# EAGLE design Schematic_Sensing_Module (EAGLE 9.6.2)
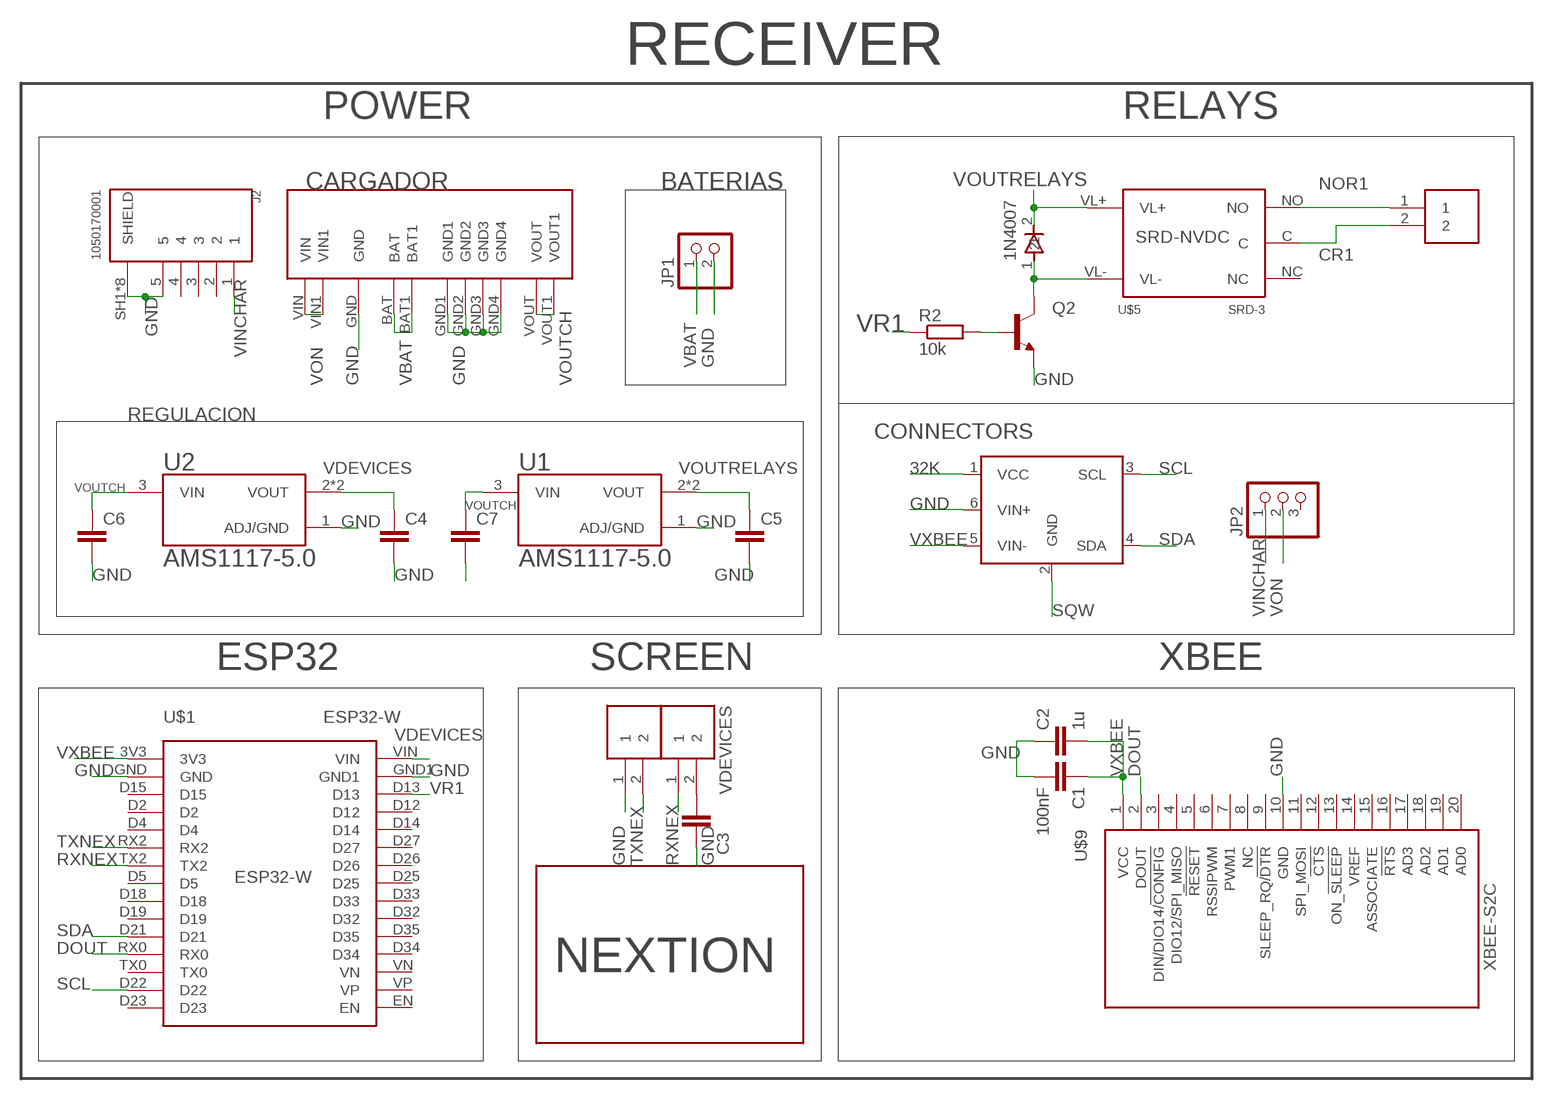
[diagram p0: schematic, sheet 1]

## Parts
1N4007  1N4007SMA  [SMA]
C1  100nF  C-EUC1206  [C1206]
C2  1u  C-EUC1206  [C1206]
C3  100nF  C-EUC1206  [C1206]
C4  C-EUC1206  [C1206]
C5  C-EUC1206  [C1206]
C6  C-EUC1206  [C1206]
C7  C-EUC1206  [C1206]
CARGADOR  MODULO_CARGA_5V  [MODULO_CARGA_5V]
CONN1  TERMINAL-TB2  [TERMINAL-TB2]
CONN2  TERMINAL-TB2  [TERMINAL-TB2]
J2  1050170001  [MOLEX_1050170001]
JP1  PINHD-1X2  [1X02]
JP2  PINHD-1X3  [1X03]
Q2  MMBT2222A  [SOT23]
R2  10k  R-EU_R1206  [R1206]
REL1  TERMINAL-TB2  [TERMINAL-TB2]
U1  AMS1117-5.0  [SOT229P700X180-4N]
U2  AMS1117-5.0  [SOT229P700X180-4N]
U$1  ESP32-W  [DIP]
U$2  NX4024T032  [NX4024T032]
U$3  INABB  [INA219-MODULE]
U$5  SRD-3  [SRD-N]
U$9  XBEE-S2C  [XBEE-DIP]

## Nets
32K: U$3.1(VCC)
CR1: REL1.2 U$5.C
DOUT: U$1.RX0 U$9.2(DOUT)
GND: C1.2 C2.1 C3.2 C4.2 C5.2 C6.2 C7.2 CARGADOR.GND CARGADOR.GND1 CARGADOR.GND2 CARGADOR.GND3 CARGADOR.GND4 CONN1.1 J2.5 J2.SH1(SHIELD) J2.SH2(SHIELD) J2.SH3(SHIELD) J2.SH4(SHIELD) J2.SH5(SHIELD) J2.SH6(SHIELD) J2.SH7(SHIELD) J2.SH8(SHIELD) JP1.2 Q2.2(E) U1.1(ADJ/GND) U2.1(ADJ/GND) U$1.GND U$1.GND1 U$3.6(VIN+) U$9.10(GND)
N$5: Q2.1(B) R2.2
N$8: 1N4007.1 Q2.3(C) U$5.VL-
NOR1: REL1.1 U$5.NO
RXNEX: CONN2.1 U$1.TX2
SCL: U$1.D22 U$3.3(SCL)
SDA: U$1.D21 U$3.4(SDA)
SQW: U$3.2(GND)
TXNEX: CONN1.2 U$1.RX2
VBAT: CARGADOR.BAT CARGADOR.BAT1 JP1.1
VDEVICES: C3.1 C4.1 CONN2.2 U2.2(VOUT) U2.4(VOUT) U$1.VIN
VINCHAR: J2.1 JP2.1
VON: CARGADOR.VIN CARGADOR.VIN1 JP2.2
VOUTCH: C6.1 C7.1 CARGADOR.VOUT CARGADOR.VOUT1 U1.3(VIN) U2.3(VIN)
VOUTRELAYS: 1N4007.2 C5.1 U1.2(VOUT) U1.4(VOUT) U$5.VL+
VR1: R2.1 U$1.D13
VXBEE: C1.1 C2.2 U$1.3V3 U$3.5(VIN-) U$9.1(VCC)
Unconnected: J2.2 J2.3 J2.4 JP2.3 U$1.D2 U$1.D4 U$1.D5 U$1.D12 U$1.D14 U$1.D15 U$1.D18 U$1.D19 U$1.D23 U$1.D25 U$1.D26 U$1.D27 U$1.D32 U$1.D33 U$1.D34 U$1.D35 U$1.EN U$1.TX0 U$1.VN U$1.VP U$5.NC U$9.3(DIN/DIO14/!CONFIG) U$9.4(DIO12/SPI_MISO) U$9.5(!RESET) U$9.6(RSSIPWM) U$9.7(PWM1) U$9.8(NC) U$9.9(SLEEP_RQ/!DTR) U$9.11(SPI_MOSI) U$9.12(!CTS) U$9.13(ON_!SLEEP) U$9.14(VREF) U$9.15(ASSOCIATE) U$9.16(!RTS) U$9.17(AD3) U$9.18(AD2) U$9.19(AD1) U$9.20(AD0)

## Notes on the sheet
- RECEIVER
- POWER | RELAYS
- BATERIAS
- REGULACION
- CONNECTORS
- ESP32 | SCREEN | XBEE

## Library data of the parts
1N4007 = 1n400X:1N4007SMA
C1-C7 = rcl:C-EU: CAPACITOR, European symbol; SPICEPREFIX: C
CARGADOR = Modulo_Carga:MODULO_CARGA_5V
CONN1 CONN2 REL1 = TERMINAL-TB001:TERMINAL-TB2
J2 = 1050170001_MOLEX:1050170001: Conn.; Data; USB; Recept.; Micro; B Type; Bottom Mount, SMT, with Solder Tabs, Lead-Free Check prices; AVAILABILITY: Warning; DESCRIPTION: USB - micro B USB 2.0 Receptacle Connector 5 Position Surface Mount, Right Angle; Through Hole; MF: Molex; MP: 1050170001; PACKAGE: None; PRICE: None; PURCHASE-URL: https://pricing.snapeda.com/search/part/1050170001/?ref=eda
JP1 = pinhead:PINHD-1X2: PIN HEADER
JP2 = pinhead:PINHD-1X3: PIN HEADER
Q2 = MMBT2222A:MMBT2222A: 2N2222 General Purpose NPN Transistor Check prices; AVAILABILITY: Good; DESCRIPTION: Bipolar (BJT) Transistor NPN 40V 600mA 300MHz 225mW Surface Mount SOT-23; MF: ON Semiconductor; MP: MMBT2222A; PACKAGE: None; PRICE: None
R2 = rcl:R-EU_: RESISTOR, European symbol; SPICEPREFIX: R
U1 U2 = AMS1117-5.0:AMS1117-5.0: Sot223/Pkg 1-Amp 5-Volt Low Drop Out Voltage Regulatator; AVAILABILITY: Unavailable; DESCRIPTION: Sot223/Pkg 1-Amp 5-Volt Low Drop Out Voltage Regulatator; MF: Advanced Monolithic Systems; MP: AMS1117-5.0; PACKAGE: None; PRICE: None
U$1 = ESP32-W:ESP32-W
U$2 = NEXTION:NX4024T032
U$3 = INA219BB:INABB
U$5 = RELE-SRD:SRD-3
U$9 = XBEES2:XBEE-S2C

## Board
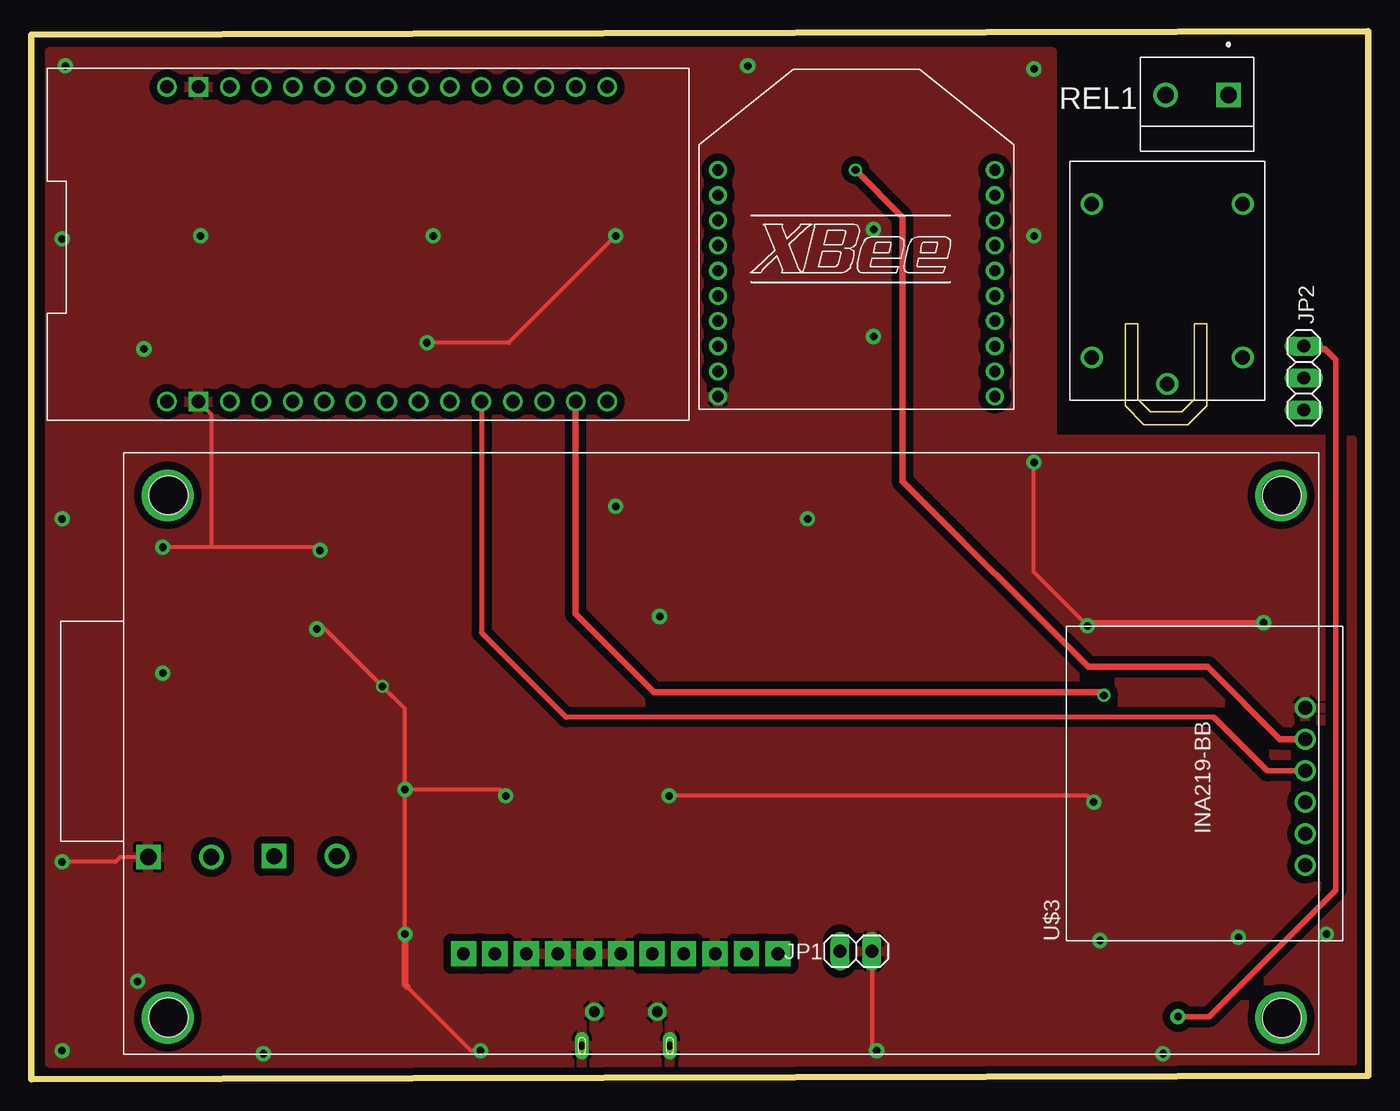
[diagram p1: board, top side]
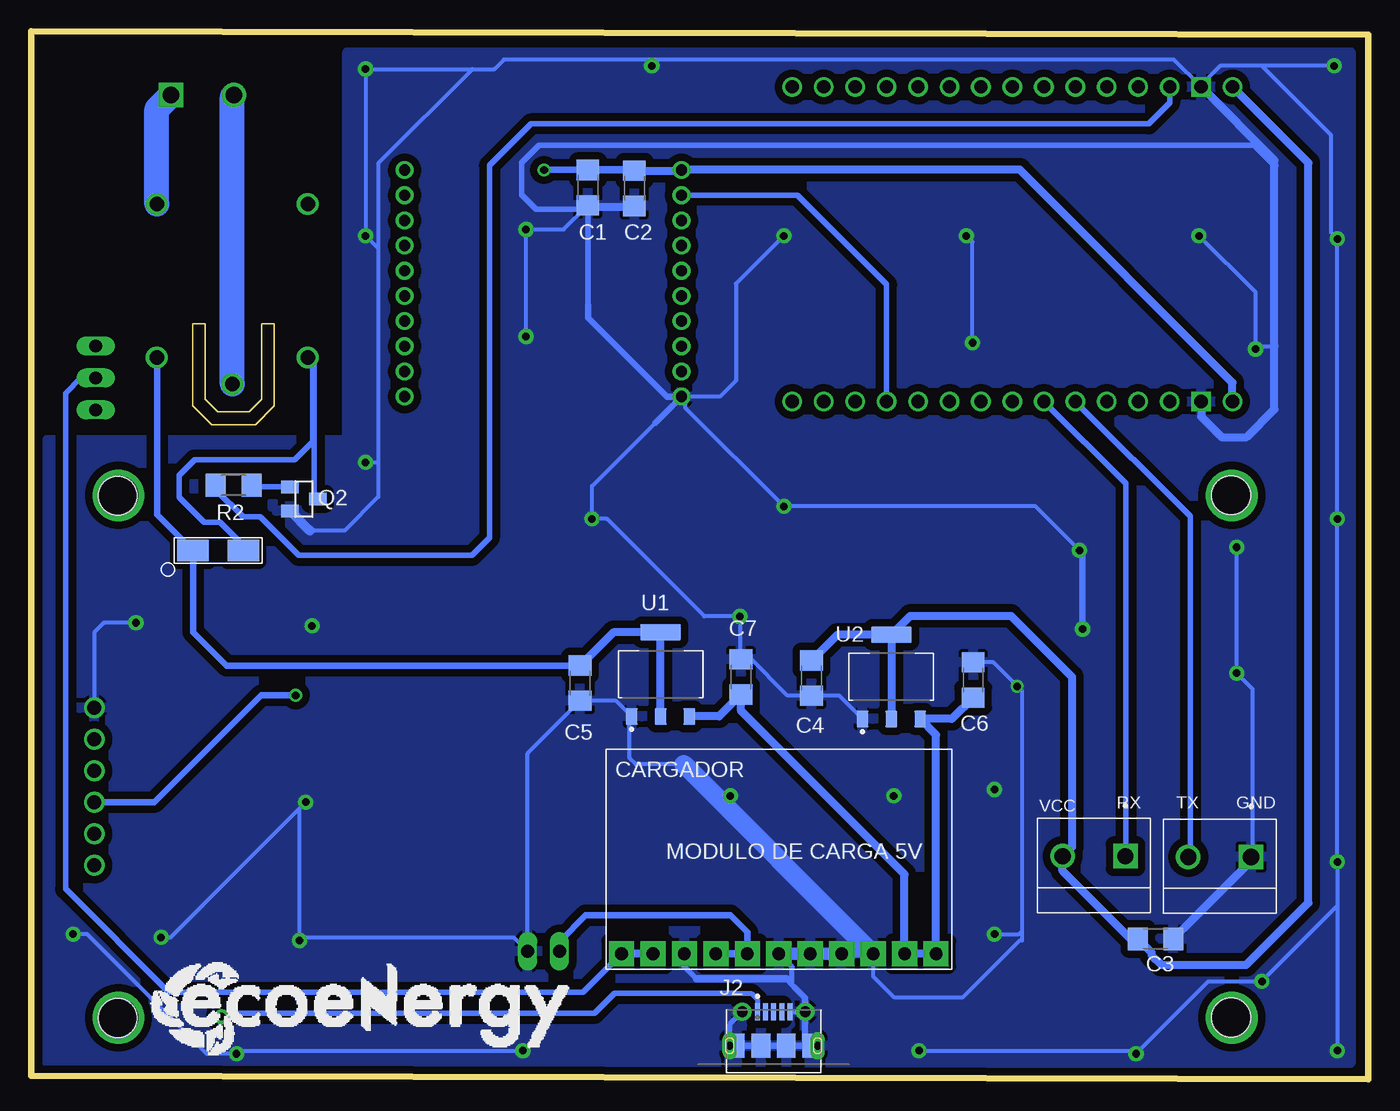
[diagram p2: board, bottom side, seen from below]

Size 106.25 x 83.25 mm. Coordinates in mm from the lower left corner, seen from the top.
Outline: 0,83 0,0 106.25,0.25 106.25,83.25 0,83
Copper layers (1*16): Top 0.035mm / dielectric 1.5mm / Bottom 0.035mm
Design rules "default *": minimum track width 0.3mm, minimum drill 0.6mm, track to track 0.6mm, track to pad 0.6mm, pad to pad 0.6mm, via to via 0.6mm, smd to smd 0.6mm, copper to edge 0.6mm, drill to drill 0.8mm, minimum pad ring 10mil, minimum via ring 8mil, stop-mask expansion 10mil, vias tented up to drill 0mil, thermal gap 10mil
Holes 3.1 mm at 10.9,46.4 10.9,4.9 99.4,4.85 99.4,46.35
Milling: 12 lines

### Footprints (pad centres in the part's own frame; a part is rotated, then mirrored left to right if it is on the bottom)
SMA = smd 2.5 x 1.7: 1 -2,0; 2 2,0
C1206 = smd 1.6 x 1.8: 1 -1.4,0; 2 1.4,0
MODULO_CARGA_5V = drill 1 pad 2 square: BAT -5,-7.5; BAT1 -2.5,-7.5; GND -7.5,-7.5; GND1 0,-7.5; GND2 2.5,-7.5; GND3 5,-7.5; GND4 7.5,-7.5; VIN -12.5,-7.5; VIN1 -10,-7.5; VOUT 10,-7.5; VOUT1 12.5,-7.5
TERMINAL-TB2 = drill 1.3 square: 1 -2.5,0 | drill 1.3: 2 2.5,0
MOLEX_1050170001 = smd 0.4 x 1.35: 1 -1.3,2.35; 2 -0.65,2.35; 3 0,2.35; 4 0.65,2.35; 5 1.3,2.35 | drill 0.85 pad 1.45: SH1 -2.5,2.35; SH2 2.5,2.35 | drill 0.6 pad 0.95 long: SH3 -3.5,-0.35; SH8 3.5,-0.35 | smd 1.2 x 1.9: SH4 -2.9,-0.35; SH7 2.9,-0.35 | smd 1.5 x 1.9: SH5 -1,-0.35; SH6 1,-0.35
1X02 = drill 1.016 long: 1 -1.27,0; 2 1.27,0
1X03 = drill 1.016 long: 1 -2.54,0; 2 0,0; 3 2.54,0
SOT23 = smd 1 x 1.4: 1 -0.95,-1.1; 2 0.95,-1.1; 3 0,1.1
R1206 = smd 1.6 x 1.803: 1 -1.422,0; 2 1.422,0
SOT229P700X180-4N = smd 0.93 x 1.31: 1 -2.29,-3.345; 2 0,-3.345; 3 2.29,-3.345 | smd 3.24 x 1.31: 4 0,3.345
DIP = drill 1.04: 3V3 12,-19; D2 12,-11.5; D4 12,-9; D5 12,-1.5; D12 -13,-11.5; D13 -13,-14; D14 -13,-9; D15 12,-14; D18 12,1; D19 12,3.5; D21 12,6; D22 12,13.5; D23 12,16; D25 -13,-1.5; D26 -13,-4; D27 -13,-6.5; D32 -13,3.5; D33 -13,1; D34 -13,8.5; D35 -13,6; EN -13,16; RX0 12,8.5; RX2 12,-6.5; TX0 12,11; TX2 12,-4; VIN -13,-19; VN -13,11; VP -13,13.5 | drill 1.04 square: GND 12,-16.5; GND1 -13,-16.5
NX4024T032 = drill 3.1: P$1 -44.5,21; P$2 -44.5,-20.5; P$3 44,21; P$4 44,-20.5
INA219-MODULE = drill 1.1: 1 -6.5,-8; 2 -4,-8; 3 -1.5,-8; 4 1,-8; 5 3.5,-8; 6 6,-8
SRD-N = drill 1.15: C 8.2,0; NC -6.1,-6; NO -6.1,6; VL+ 6.1,6; VL- 6.1,-6
XBEE-DIP = drill 0.9: 1 -11,9; 2 -11,7; 3 -11,5; 4 -11,3; 5 -11,1; 6 -11,-1; 7 -11,-3; 8 -11,-5; 9 -11,-7; 10 -11,-9; 11 11,-9; 12 11,-7; 13 11,-5; 14 11,-3; 15 11,-1; 16 11,1; 17 11,3; 18 11,5; 19 11,7; 20 11,9

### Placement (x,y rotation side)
1N4007  91.4,42 180 bottom
C1  62.01,70.84 270 bottom
C2  58.32,70.78 90 bottom
C3  16.89,11.14 0 bottom
C4  44.24,31.86 270 bottom
C5  62.64,31.46 270 bottom
C6  31.39,31.71 90 bottom
C7  49.84,31.96 90 bottom
CARGADOR  46.84,17.46 0 bottom
CONN1  11.79,17.66 180 bottom
CONN2  21.79,17.71 180 bottom
J2  47.25,3 0 bottom
JP1  65.54,10.16 0 top
JP2  101.14,55.71 270 top
Q2  84.59,46.1 270 bottom
R2  90.18,47.19 0 bottom
REL1  92.65,78.21 180 top
U1  56.24,32.16 0 bottom
U2  37.89,31.96 0 bottom
U$1  29.77,65.84 270 top
U$2  54.83,25.88 180 top
U$3  93.25,23.5 90 top
U$5  90.29,63.43 270 top
U$9  65.58,63.23 0 top

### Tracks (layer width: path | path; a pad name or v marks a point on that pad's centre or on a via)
CR1
  Bottom 2: U$5.C 90.29,78.07 REL1.2
DOUT
  Bottom 0.45: U$1.RX0 38.27,63.14 45.36,70.23 U$9.2
GND  (via drill 0.6, 0.6 pad 1.2)
  Top 0.3: U$1.GND 14.27,52.84 14.27,42.34 14.19,42.26 v10.44,42.26 22.69,42.26 v22.94,42.01 | v46.44,67.01 37.94,58.51 v31.44,58.51 | CONN1.1 7.09,17.66 6.69,17.26 v2.44,17.26 | v35.69,2.26 34.94,2.26 29.85,7.35 | v29.69,11.51 v29.69,23.01 | v29.69,23.01 37.19,23.01 v37.69,22.51 | v29.69,23.01 29.69,29.41 v27.89,31.21 23.34,35.76 v22.69,35.76 | v84.44,22.01 83.94,22.51 v50.69,22.51 | v67.19,2.26 66.81,2.64 JP1.2 | v83.94,36.01 83.73,36.23 79.69,40.26 v79.69,49.01
  Top 0.5: v97.94,36.26 97.91,36.23 83.73,36.23 | 29.85,7.35 29.69,7.51 v29.69,11.51
  Bottom 0.3: CARGADOR.GND 54.59,9.71 54.59,9.15 | 54.39,25.01 58.19,25.01 58.69,25.51 58.69,28.66 U1.1 59.78,30.06 C5.2 66.81,25.89 JP1.2 67.91,11.26 84.69,11.26 v84.94,11.01 84.94,21.51 v84.44,22.01 95.19,11.26 v95.94,11.26 | U2.1 42.03,30.46 C4.2 46.14,30.46 49.19,33.51 49.69,33.51 C7.2 49.94,33.46 v49.94,36.76 52.76,36.76 60.51,44.51 v61.69,44.51 61.69,47.12 56.66,52.16 | CARGADOR.GND4 39.34,8.16 37.69,6.51 32.19,6.51 27.7,11 27.5,11 27.5,11.75 | 56.75,81.01 15.44,81.01 U$1.GND1 13.27,79 11.76,80.51 8.44,80.51 | 56.75,81.01 68.69,81.01 69.44,80.26 71.19,80.26 | 78.69,66.01 78.69,72.76 71.19,80.26 | 78.69,66.01 v79.69,67.01 v79.69,80.26 71.19,80.26 | 78.69,66.01 78.69,49 | 78.69,49 78.69,46.26 81.37,43.59 84.13,43.59 | v67.19,2.26 89.69,2.26 v89.94,2.01 92.32,2.01 101.82,11.51 v102.94,11.51 | v35.69,2.26 18.69,2.26 v18.44,2.01 12.69,7.76 v8.44,7.76 2.44,13.76 v2.44,17.26 | v2.44,17.26 v2.44,2.26 | v2.44,17.26 v2.44,44.51 v2.44,66.76 2.94,67.26 2.94,75.01 8.44,80.51 | v2.69,80.51 8.44,80.51 | v13.44,67.01 8.94,62.51 v8.94,58.01 8.71,58.25 7.44,58.25 | v31.44,58.51 31.44,66.51 v31.94,67.01 | v46.44,67.01 50.25,63.2 50.25,55.5 51.52,54.23 54.25,54.23 | 54.25,54.23 U$9.10 | 54.25,54.23 54.25,53.32 v46.44,45.51 26.44,45.51 v22.94,42.01 | v66.94,59.01 v66.94,67.51 63.94,67.51 C1.2 | v56.94,80.51 56.75,80.7 56.75,81.01 | v10.44,42.26 v10.44,32.26 9.19,31.01 9.19,17.56 CONN1.1 | v79.69,49.01 78.7,49.01 78.69,49 | v97.94,36.26 100.49,36.26 101.25,35.5 U$3.6 | 27.5,11.75 27.5,30.82 v27.89,31.21 29.79,33.11 C6.2 | v29.69,11.51 27.74,11.51 27.5,11.75
  Bottom 0.4: 45.79,7.51 45.79,8.91 CARGADOR.GND1 | 53.4,7.96 54.59,9.15 | 45.54,7.26 45.79,7.51 | 45.79,7.51 46.24,7.96 | J2.5 45.1,5.35 44.75,5 | J2.SH1 50.75,4.35 J2.SH3
  Bottom 0.45: 62.01,61.5 62.01,69.11 | 62.01,69.11 C1.2 | 7.44,72.61 9.04,74.21 65.89,74.21 67.29,72.81 67.29,70.26 66.14,69.11 62.01,69.11
  Bottom 0.5: 56.66,52.16 U$9.10 55.73,54.23 62.01,60.51 62.01,61.5 | v22.69,35.76 22.69,41.76 v22.94,42.01 | J2.SH4 J2.SH5 J2.SH6 J2.SH7 44.75,3.05 44.75,5 J2.SH2 44.75,6.47 45.54,7.26
  Bottom 0.6: 46.24,7.96 53.4,7.96
  Bottom 0.65: CARGADOR.GND4 CARGADOR.GND3 | C3.2 9.29,17.34 CONN1.1 | C1.2 61.88,69.31 58.39,69.31 C2.1 | U$1.GND 13.27,52.64 11.64,51.01 9.64,51.01 7.44,53.21 7.44,58.25 7.44,72.61 7.44,73.01 U$1.GND1
  Bottom 0.8: 84.13,43.59 Q2.2
  Bottom 1: CARGADOR.GND3 CARGADOR.GND2 CARGADOR.GND1
  Bottom 1.5: CARGADOR.GND4 54.39,25.01
  pour Bottom (isolate 0.6): 81.14,81.61 1.39,81.61 1.39,1.26 104.99,1.26 104.99,50.81 81.14,50.81
  pour Top (isolate 0.6): 104.99,1.31 104.99,50.81 81.14,50.81 81.14,81.61 1.44,81.61 1.44,1.31
N$5
  Bottom 0.45: Q2.1 88.62,47.05 R2.2
N$8
  Bottom 0.45: Q2.3 83.79,46.4 83.79,56.83 U$5.VL- 83.89,56.93 83.89,50.66 85.34,49.21 93.29,49.21 94.5,48 94.5,46.25 92.5,44.25 91.25,44.25 89.4,42.4
  Bottom 0.5: 1N4007.1 89.4,42.4
NOR1
  Bottom 2: U$5.NO 96.29,77.07 REL1.1
RXNEX
  Bottom 0.45: U$1.TX2 19.27,47.34 19.27,17.73 CONN2.1
SCL  (via drill 0.6)
  Top 0.5: U$1.D22 43.27,36.98 49.5,30.75 85,30.75 v85.25,30.5
  Bottom 0.5: v85.25,30.5 88,30.5 96.5,22 U$3.3
SDA
  Top 0.4: U$1.D21 35.77,35.48 42.5,28.75 94,28.75
  Top 0.45: U$3.4 98.25,24.5 94,28.75
TXNEX
  Bottom 0.45: CONN1.2 14.14,17.81 14.14,44.71 U$1.RX2
VBAT
  Bottom 0.5: CARGADOR.BAT1 49.34,11.66 50.69,13.01 62.19,13.01 64.19,11.01 64.19,10.24
  Bottom 0.6: 64.19,10.24 JP1.1 | CARGADOR.BAT CARGADOR.BAT1
VDEVICES
  Bottom 0.65: U2.4 U2.2 | U2.4 42.2,35.31 C4.1 | U2.4 36.39,36.81 28.39,36.81 23.54,31.96 23.54,18.46 CONN2.2 24.29,16.54 18.89,11.14 C3.1 17.22,10.07 17.22,9.86 16.42,9.07 9.69,9.07 4.74,14.01 4.74,72.81 U$1.VIN
VINCHAR  (via drill 0.6 pad 1.2)
  Top 0.45: v91.14,4.96 93.64,4.96 103.69,15.01 103.69,57.16 102.85,58
  Top 0.5: 102.85,58 101.39,58 JP2.1
  Bottom 0.4: 50.44,6.81 49.01,6.81 48.55,6.35 J2.1
  Bottom 0.45: 50.44,6.81 59.89,6.81 61.49,5.21 90.89,5.21 v91.14,4.96
VON
  Bottom 0.45: CARGADOR.VIN 62.39,6.91 95.34,6.91 103.54,15.11 103.54,54.51 102.34,55.71 JP2.2
  Bottom 0.65: CARGADOR.VIN1 CARGADOR.VIN
VOUTCH
  Bottom 0.65: U1.3 51.59,28.82 C7.1 49.84,29.26 36.84,16.26 CARGADOR.VOUT CARGADOR.VOUT1 34.34,27.36 U2.3 33.09,28.62 C6.1
VOUTRELAYS
  Bottom 0.5: C5.1 90.75,32.86 93.4,35.52 1N4007.2 96.25,44.84 96.25,57.29 U$5.VL+
  Bottom 0.65: U1.2 U1.4 60,35.51 C5.1
VR1
  Bottom 0.3: R2.1 91.6,46.84
  Bottom 0.45: U$1.D13 15.77,77.58 17.44,75.91 66.54,75.91 69.84,72.61 69.84,43.01 71.24,41.61 85,41.61 88.06,44.67 89.44,44.67 91.6,46.84
VXBEE  (via drill 0.6)
  Top 0.5: v65.5,72.25 69.25,68.5 69.25,47.5 84,32.75 93.5,32.75 99.25,27 U$3.5
  Bottom 0.45: 58.38,72.24 C2.2
  Bottom 0.5: v65.5,72.25 v65.49,72.24 C1.1
  Bottom 0.6: C1.1 58.38,72.24
  Bottom 0.65: U$1.3V3 10.77,55.34 27.69,72.26 54.55,72.26 U$9.1 54.63,72.18 C2.2

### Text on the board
bPlace: VCC | GND | TX | RX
